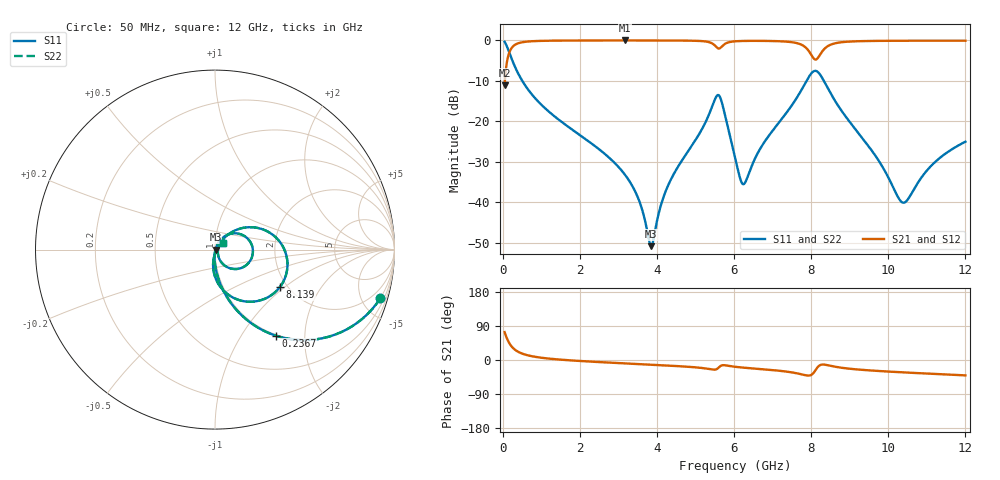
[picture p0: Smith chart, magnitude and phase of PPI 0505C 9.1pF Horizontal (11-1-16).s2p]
# MHz S MA R 50
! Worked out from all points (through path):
!   1601 points, 50 MHz to 12 GHz, reference 50 ohm
!   highest |S21| = -0.02 dB at 3.179 GHz (marker M1); lowest = -11.1 dB at 50 MHz (marker M2)
!   group delay of S21, straight-line fit = 12 ps
!   lowest |S11| = -50.8 dB at 3.852 GHz (marker M3), VSWR 1.01, Z = 50.3 - j0.0701 ohm
!   |S11| at or under -10 dB: 508.1 MHz to 7.881 GHz (7.373 GHz wide, 176 % of centre); 8.329 GHz to end of sweep
!   |S22| runs from -50.8 to -0.4 dB; largest |S21 - S12| = 0
!   S11 on the Smith chart (normalised r, x): 50 MHz: 0.98, -6.80; 236.7 MHz: 0.98, -1.43; 8.139 GHz: 1.83, -0.92; 12 GHz: 1.08, +0.08
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50  0.9601 -16.4  0.2797 73.6  0.2797 73.6  0.9601 -16.4
236.7188  0.5857 -54.9  0.8099 35.1  0.8099 35.1  0.5857 -54.9
647.5  0.2511 -77.3  0.9669 12.4  0.9669 12.4  0.2511 -77.3
2044.156  0.06548 -91.3  0.996 -2.9  0.996 -2.9  0.06548 -91.3
3179.406  0.02168 -93.0  0.9973 -9.0  0.9973 -9.0  0.02168 -93.0
3530.438  0.01075 -87.1  0.9972 -10.8  0.9972 -10.8  0.01075 -87.1
3851.594  0.002878 -14.0  0.9969 -12.4  0.9969 -12.4  0.002878 -14.0
4038.312  0.00705 50.1  0.9966 -13.4  0.9966 -13.4  0.00705 50.1
4359.469  0.01902 63.1  0.9956 -15.1  0.9956 -15.1  0.01902 63.1
5561.938  0.2089 3.9  0.8093 -23.3  0.8093 -23.3  0.2089 3.9
5688.906  0.168 -39.5  0.8454 -14.1  0.8454 -14.1  0.168 -39.5
6025  0.03602 -60.9  0.973 -17.9  0.973 -17.9  0.03602 -60.9
6278.938  0.01729 5.8  0.9841 -20.5  0.9841 -20.5  0.01729 5.8
6704.656  0.04819 50.5  0.9856 -24.1  0.9856 -24.1  0.04819 50.5
7451.531  0.1465 44.7  0.9555 -31.9  0.9555 -31.9  0.1465 44.7
8019.156  0.3985 -4.5  0.6435 -38.3  0.6435 -38.3  0.3985 -4.5
8138.656  0.4174 -30.0  0.584 -22.9  0.584 -22.9  0.4174 -30.0
8594.25  0.1874 -85.0  0.9134 -17.2  0.9134 -17.2  0.1874 -85.0
10013.31  0.01978 -85.0  0.9877 -30.6  0.9877 -30.6  0.01978 -85.0
10431.56  0.01002 -20.0  0.9896 -32.9  0.9896 -32.9  0.01002 -20.0
11148.56  0.02939 37.2  0.9906 -36.5  0.9906 -36.5  0.02939 37.2
12000  0.05608 41.7  0.9902 -40.6  0.9902 -40.6  0.05608 41.7
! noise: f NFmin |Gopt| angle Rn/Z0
50  0.0004786  0.8925  1.487  0.0009704
1372  0.004474  0.7045  4.842  0.002966
2701  0.007483  0.6617  8.909  0.004207
4031  0.01136  0.6676  12.95  0.006481
5360  0.04972  0.8864  17.14  0.09298
6682  0.02914  0.7743  21.25  0.0255
8012  0.194  0.9556  25.42  0.9356
9341  0.04129  0.7805  29.6  0.03609
1.067e+04  0.03088  0.6859  33.43  0.01755
1.2e+04  0.02976  0.6461  37.08  0.0144
